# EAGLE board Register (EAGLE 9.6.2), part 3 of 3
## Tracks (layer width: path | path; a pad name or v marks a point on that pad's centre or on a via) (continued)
N$147  (via drill 0.35) (continued)
  Top 0.152: 87.01,49.94 87.01,46.2 87.19,46.03 89.32,46.03 90.03,46.74 90.03,47.27 IC66.3 | 87.01,49.94 89.32,52.25 90.74,52.25 91.27,52.78 91.27,53.49 IC66.13 | v17.84,44.07 17.84,42.47 IC27.11 | v65.49,45.49 68.87,45.49 69.05,45.31 71.89,45.31 75.45,48.87 77.58,48.87 78.3,48.16 78.3,47.45 IC65.3 78.3,47.27 77.76,46.74 v77.76,45.85 | v78.12,51.18 79.54,52.6 79.54,53.49 IC65.13 | v85.41,49.94 87.01,49.94
  Route2 0.152: v17.84,44.07 17.84,42.82 21.4,39.27 25.49,39.27 29.04,42.82 62.83,42.82 v65.49,45.49
  Route3 0.152: v85.41,49.94 79.36,49.94 v78.12,51.18
  Bottom 0.152: v78.12,51.18 78.12,46.2 v77.76,45.85
N$148  (via drill 0.35)
  Top 0.152: v27.09,34.65 26.38,35.36 26.38,36.25 IC111.2 | v97.32,66.12 94.83,66.12 94.12,65.41 94.12,64.69 IC56.11
  Route14 0.152: v27.09,34.65 27.44,34.65 43.98,51.18 50.38,51.18 64.78,65.58 96.79,65.58 v97.32,66.12
N$149  (via drill 0.35)
  Top 0.152: v30.29,34.65 29.93,34.65 29.04,35.53 29.04,36.25 IC111.4 | v80.07,55.98 90.21,55.98 91.45,57.23 91.99,57.23 92.7,57.94 92.7,58.47 IC56.5
  Route3 0.152: v30.29,34.65 46.82,51.18 56.96,51.18 58.2,52.43 62.83,52.43 66.03,55.63 79.72,55.63 v80.07,55.98
N$150  (via drill 0.35)
  Top 0.152: v31.36,34.65 31.36,36.25 IC111.6 | v82.56,61.14 82.56,64.34 IC55.11
  Route14 0.152: v31.36,34.65 37.05,34.65 60.69,58.29 73.85,58.29 76.7,61.14 v82.56,61.14
N$151  (via drill 0.35)
  Top 0.152: v32.6,45.14 32.6,42.47 IC111.10 | v78.3,60.43 79.54,60.43 80.96,59 IC55.5
  Route2 0.152: v32.6,45.14 34.73,47.27 34.73,47.45 48.25,60.96 58.38,60.96 61.05,58.29 76.16,58.29 v78.3,60.43
N$156  (via drill 0.35)
  Top 0.152: v76.87,60.25 75.98,59.36 75.98,58.65 IC55.1 | v93.76,60.25 96.61,60.25 98.92,57.94 98.92,57.4 99.1,57.23 100.16,57.23 100.88,57.94 100.88,58.47 IC58.2
  Route14 0.152: v76.87,60.25 77.41,60.25 77.94,59.72 89.5,59.72 89.67,59.54 93.05,59.54 v93.76,60.25
N$157
  Top 0.152: IC56.15 88.96,64.69 88.96,65.23 90.56,66.83 100.25,66.83 100.88,66.2 100.88,64.69 IC58.13
N$158
  Top 0.152: IC56.1 87.72,58.65 87.72,59.18 90.03,61.49 103.37,61.49 106.03,64.16 106.03,64.52 IC58.9
N$159
  Top 0.152: IC58.6 106.21,58.65 106.21,61.67 107.99,63.45 107.99,65.76 106.57,67.18 78.47,67.18 77.23,65.94 77.23,64.69 IC55.15
N$160
  Top 0.152: IC98.5 44.87,3.71 44.87,4.24 47.18,6.55 62.47,6.55 64.6,8.69 64.6,9.58 IC97.13
N$161  (via drill 0.35)
  Top 0.152: 50.74,48.51 50.74,46.2 50.91,46.03 53.23,46.03 53.94,46.74 53.94,47.27 IC61.3 | 50.74,48.51 55.18,52.96 55.18,53.49 IC61.13 | v22.47,38.2 19.09,38.2 17.84,36.96 17.84,36.42 IC27.4 | v35.45,44.42 35.45,44.96 39.36,48.87 41.31,48.87 42.2,47.98 42.2,47.45 IC60.3 | v42.2,51.18 43.45,52.43 43.45,53.49 IC60.13 | v49.49,48.51 50.74,48.51
  Route2 0.152: v49.49,48.51 44.87,48.51 v42.2,51.18
  Route3 0.152: v22.47,38.2 23.36,38.2 28.69,43.54 34.56,43.54 v35.45,44.42
  Bottom 0.152: v35.45,44.42 v42.2,51.18
N$162  (via drill 0.35)
  Top 0.152: v38.29,31.45 38.29,31.09 34.38,27.18 33.13,27.18 31.53,25.58 31.53,24.87 IC110.6 | v58.56,51.71 58.56,52.25 57.85,52.96 57.85,53.49 IC61.11
  Route3 0.152: v58.56,51.71 v38.29,31.45
N$163  (via drill 0.35)
  Top 0.152: v32.78,32.69 32.78,31.09 IC110.10 | v49.31,45.85 50.56,45.85 50.74,45.67 55.36,45.67 56.43,46.74 56.43,47.27 IC61.5
  Bottom 0.152: v32.78,32.69 32.78,33.58 45.05,45.85 v49.31,45.85
N$164  (via drill 0.35)
  Top 0.152: v29.22,29.31 30.11,30.2 30.11,30.91 IC110.12 | v44.51,51.89 44.87,51.89 45.94,52.96 45.94,53.49 IC60.11
  Route3 0.152: v29.22,29.31 29.22,36.6 v44.51,51.89
N$165
  Top 0.152: IC110.15 26.38,31.09 26.38,31.62 28.69,33.93 31.71,33.93 32.07,34.29 32.07,39.98 33.31,41.22 33.31,48.51 34.38,49.58 43.09,49.58 44.69,47.98 44.69,47.45 IC60.5
N$170
  Top 0.152: IC60.1 39.71,47.27 39.71,46.74 41.31,45.14 55.88,45.14 56.78,46.04 59.42,46.04 60.33,45.14 63,45.14 64.6,46.74 64.6,47.27 IC63.2
N$171
  Top 0.152: IC61.15 52.87,53.67 52.87,54.2 53.94,55.27 63.54,55.27 64.6,54.2 64.6,53.67 IC63.13
N$172
  Top 0.152: IC61.1 51.45,47.45 51.45,47.98 54.47,51 69.41,51 69.94,51.54 69.94,53.49 IC63.9
N$173  (via drill 0.35)
  Top 0.152: v59.09,50.11 59.45,50.47 68.16,50.47 69.76,48.87 69.76,47.45 IC63.6 | v44.51,55.27 42.02,55.27 40.96,54.2 IC60.15
  Route15 0.152: v59.09,50.11 50.03,50.11 45.58,54.56 45.22,54.56 v44.51,55.27
N$174  (via drill 0.35)
  Top 0.152: v85.23,3.53 87.54,3.53 IC99.1 | v50.38,9.04 48.43,9.04 47.71,8.33 46.82,8.33 46.11,9.04 46.11,9.58 IC98.9
  Route2 0.152: v85.23,3.53 61.4,3.53 58.03,6.91 53.94,6.91 51.8,9.04 v50.38,9.04
N$175  (via drill 0.35)
  Top 0.152: v87.01,60.96 87.01,57.23 89.5,57.23 90.03,57.76 90.03,58.47 IC56.3 | IC56.13 91.27,64.52 91.27,63.98 89.5,62.2 88.43,62.2 88.07,62.56 v87.72,62.56 85.41,64.87 85.41,65.94 84.87,66.47 80.96,66.47 79.72,65.23 79.72,64.69 IC55.13 79.54,64.52 79.54,62.74 77.58,60.78 77.58,59.89 78.3,59.18 78.3,58.65 IC55.3 78.3,58.47 78.3,57.76 v76.87,56.34 | v20.87,51.18 19.62,51.18 17.84,52.96 17.84,53.49 IC24.11
  Route3 0.152: v20.87,51.18 24.24,51.18 25.67,52.6 37.76,52.6 37.93,52.43 40.25,52.43 40.6,52.78 62.65,52.78 65.85,55.98 76.52,55.98 v76.87,56.34
  Bottom 0.152: v87.01,60.96 87.01,61.85 v87.72,62.56
N$177  (via drill 0.35)
  Top 0.152: v29.76,21.31 30.11,20.96 30.11,19.71 IC109.12 | v93.97,52.21 v93.96,52.21 93.96,53.54 IC66.11
  Route15 0.152: v29.76,21.31 29.76,21.67 35.27,27.18 46.11,27.18 67.27,48.34 74.21,48.34 78.47,52.6 93.73,52.6 93.97,52.37 v93.97,52.21
N$178  (via drill 0.35)
  Top 0.152: v27.98,17.93 27.44,17.93 26.38,19 26.38,19.53 IC109.15 | v91.81,49.05 92.7,48.16 92.7,47.45 IC66.5
  Route3 0.152: v27.98,17.93 28.87,17.93 63.54,52.6 72.25,52.6 80.61,44.25 80.61,43.71 86.12,38.2 87.19,38.2 88.25,39.27 88.25,45.49 v91.81,49.05
N$179  (via drill 0.35)
  Top 0.152: v26.91,27.36 26.38,26.82 26.38,24.87 IC110.2 | v80.07,51.89 81.14,51.89 82.21,52.96 82.21,53.49 IC65.11
  Route2 0.152: v26.91,27.36 30.65,27.36 45.76,42.47 70.65,42.47 v80.07,51.89
N$180  (via drill 0.35)
  Top 0.152: v33.31,28.96 32.42,28.96 29.04,25.58 29.04,24.87 IC110.4 | v80.07,49.05 80.96,48.16 IC65.5
  Route2 0.152: v33.31,28.96 34.73,30.38 34.73,30.56 41.49,37.31 56.25,37.31 61.05,42.11 72.96,42.11 79.9,49.05 v80.07,49.05
N$185
  Top 0.152: IC65.1 75.98,47.27 75.98,46.56 77.41,45.14 99.28,45.14 100.88,46.74 100.88,47.27 IC68.2
N$186
  Top 0.152: IC66.15 88.96,53.67 88.96,54.2 90.92,56.16 99.28,56.16 100.88,54.56 100.88,53.67 IC68.13
N$187
  Top 0.152: IC66.1 87.72,47.45 87.72,50.11 88.43,50.83 103.9,50.83 106.03,52.96 106.03,53.49 IC68.9
N$188  (via drill 0.35)
  Top 0.152: v103.54,45.67 104.79,45.67 106.03,46.91 106.03,47.27 IC68.6 | v88.96,55.27 77.76,55.27 77.23,54.74 77.23,53.67 IC65.15
  Route2 0.152: v103.54,45.67 102.3,45.67 93.23,54.74 89.5,54.74 v88.96,55.27
N$189  (via drill 0.35)
  Top 0.152: v49.14,7.26 46.65,7.26 44.87,9.04 44.87,9.58 IC98.10 | v85.41,5.66 85.41,8.69 87.01,10.29 87.01,11 87.19,11.18 88.07,11.18 88.79,10.47 88.79,9.75 IC99.13
  Bottom 0.152: v49.14,7.26 50.03,7.26 53.05,4.24 67.63,4.24 67.98,3.89 83.63,3.89 v85.41,5.66
N$190  (via drill 0.35)
  Top 0.152: v77.76,1.4 78.47,0.69 94.65,0.69 97.5,3.53 99.63,3.53 IC100.1 | v40.96,5.31 40.96,6.55 43.45,9.04 43.45,9.58 IC98.11
  Bottom 0.152: v77.76,1.4 58.74,1.4 58.56,1.22 45.05,1.22 v40.96,5.31
N$191  (via drill 0.35)
  Top 0.152: IC98.12 42.22,10.94 42.46,11.18 v50.56,11.18 | v86.12,8.33 87.36,8.33 88.79,6.91 98.74,6.91 100.88,9.04 100.88,9.58 IC100.13
  Route2 0.152: v50.56,11.18 52.69,11.18 56.6,7.26 85.05,7.26 v86.12,8.33
N$192
  Top 0.152: IC98.13 40.96,8.51 35.98,3.53 OUTPUT.4
N$194  (via drill 0.35)
  Top 0.152: IC109.2 v26.35,14.61 | v57.73,43.91 57.73,43.89 57.73,43.59 57.73,42.5 IC71.11
  Route14 0.152: v35.56,20 37.99,22.43 38.56,22.43 55.24,39.1 55.24,41.14 57.73,43.64 v57.73,43.91
  Route15 0.152: v26.35,14.61 31.75,20 v35.56,20
N$195  (via drill 0.35)
  Top 0.152: v32.07,17.93 29.04,14.91 29.04,13.49 IC109.4 | v52.34,38.02 55.36,38.02 56.43,36.96 56.43,36.42 IC71.5
  Route3 0.152: v32.07,17.93 32.07,18.29 35.27,21.49 35.27,23.09 50.2,38.02 v52.34,38.02
N$196  (via drill 0.35)
  Top 0.152: v33.31,16.87 31.53,15.09 31.53,13.49 IC109.6 | v46.29,40.51 46.29,42.11 46.11,42.29 IC70.11
  Route2 0.152: v42.56,38.02 43.8,38.02 v46.29,40.51
  Bottom 0.152: v33.31,16.87 37.22,16.87 41.85,21.49 41.85,37.31 v42.56,38.02
N$197  (via drill 0.35)
  Top 0.152: v36.16,27.89 35.09,26.82 34.02,26.82 33.31,26.11 33.31,22.55 32.78,22.02 32.78,19.71 IC109.10 | v40.96,32.69 42.91,32.69 44.69,34.47 44.69,36.25 IC70.5
  Bottom 0.152: v40.96,32.69 v36.16,27.89
N$202  (via drill 0.35)
  Top 0.152: v64.96,38.56 64.96,36.6 64.78,36.42 IC73.2 | IC70.1 39.69,37.94 v39.53,38.1
  Route3 0.152: v39.53,38.1 48.18,46.75 v50.08,46.75 | v64.96,40.34 64.96,43.67 64.84,43.8 64.84,45.02 v62.51,47.35
  Route15 0.152: v50.08,46.75 61.91,46.75 v62.51,47.35
  Bottom 0.152: v64.96,38.56 v64.96,40.34
N$203
  Top 0.152: IC71.15 52.87,42.47 52.87,43.18 53.94,44.25 56.52,44.25 57.04,44.77 59.17,44.77 59.69,44.25 63.54,44.25 64.6,43.18 64.6,42.47 IC73.13
N$204
  Top 0.152: IC71.1 51.45,36.42 51.45,38.2 52.87,39.62 67.63,39.62 69.76,41.76 69.76,42.29 IC73.9
N$205
  Top 0.152: IC70.15 40.96,43 42.74,44.78 56.2,44.78 56.82,45.4 59.39,45.4 60.01,44.78 69.41,44.78 70.47,43.71 70.47,41.22 69.94,40.69 69.94,36.42 IC73.6
N$206
  Top 0.152: IC98.1 39.54,3.53 38.29,3.53 36.33,1.58 35.27,1.58 33.49,3.35 OUTPUT.3
N$208  (via drill 0.35)
  Top 0.152: v48.07,22.38 48.07,18.29 47.36,17.58 46.82,17.58 44.87,15.62 44.87,13.84 IC108.6 | v98.74,40.51 98.74,42.11 96.96,43.89 94.83,43.89 94.12,43.18 94.12,42.47 IC76.11
  Route2 0.152: v48.07,22.38 57.85,22.38 58.03,22.2 62.12,22.2 71.54,31.62 102.43,31.62 104.08,33.28 104.08,35.17 v98.74,40.51
N$209  (via drill 0.35)
  Top 0.152: v45.76,18.29 45.94,18.47 45.94,19.89 IC108.10 | v92.16,38.02 92.21,38.02 92.71,37.52 IC76.5
  Route15 0.152: v45.76,18.29 64.78,37.31 91.45,37.31 v92.16,38.02
N$210  (via drill 0.35)
  Top 0.152: v43.45,21.67 43.45,20.07 IC108.12 | v77.58,38.56 78.83,38.56 82.21,41.94 82.21,42.29 IC75.11
  Route15 0.152: v43.45,21.67 45.4,21.67 50.74,27 50.74,27.53 61.05,37.85 76.87,37.85 v77.58,38.56
N$211  (via drill 0.35)
  Top 0.152: v39.89,21.67 39.71,21.49 39.71,20.07 IC108.15 | v80.07,38.02 80.07,37.67 80.96,36.78 IC75.5
  Route14 0.152: v39.89,21.67 60.34,42.11 75.45,42.11 79.54,38.02 v80.07,38.02
N$216
  Top 0.152: IC75.1 75.98,36.25 75.98,35.71 77.76,33.93 99.63,33.93 100.88,35.18 100.88,36.25 IC78.2
N$217
  Top 0.152: IC76.15 88.96,42.47 88.96,43 90.21,44.25 99.81,44.25 100.88,43.18 100.88,42.47 IC78.13
N$218
  Top 0.152: IC76.1 87.72,36.42 87.72,36.96 90.03,39.27 103.37,39.27 106.03,41.94 106.03,42.29 IC78.9
N$219  (via drill 0.35)
  Top 0.152: v77.76,40.87 77.23,41.4 77.23,42.29 IC75.15 | v105.14,38.02 106.03,37.14 106.03,36.42 IC78.6
  Route2 0.152: v77.76,40.87 89.32,40.87 89.85,41.4 101.77,41.4 v105.14,38.02
N$220  (via drill 0.35)
  Top 0.152: v52.16,7.62 52.69,8.15 52.69,9.58 IC92.13
  Route2 0.152: v52.16,7.62 50.91,7.62 47.89,4.6 31.89,4.6 30.82,3.53 OUTPUT.2
N$222
  Top 0.152: IC22.15 51.45,20.07 51.45,20.42 53.4,22.38 56.07,22.38 57.14,23.44 57.14,30.38 57.67,30.91 IC81.11
N$223  (via drill 0.35)
  Top 0.152: IC81.5 56.52,23.84 55.94,23.27 v55.89,23.27 | IC108.2 v39.69,12.41
  Route2 0.152: v46.65,16.33 42.38,20.6 42.38,23.62 42.91,24.16 55,24.16 v55.89,23.27
  Route3 0.152: v39.69,12.41 41.14,13.86 41.14,15.56 41.92,16.33 v46.65,16.33
N$224  (via drill 0.35)
  Top 0.152: v46.11,32.69 46.11,31.09 IC80.11 | v58.38,22.91 58.38,20.6 57.85,20.07 IC22.10
  Route2 0.152: v51.45,27.18 54.11,27.18 v58.38,22.91
  Bottom 0.152: v46.11,32.69 51.45,27.36 v51.45,27.18
N$225  (via drill 0.35)
  Top 0.152: IC108.4 42.2,13.84 42.2,12.49 v42.18,12.47 | IC80.5 44.69,24.87 44.69,23.27 44.45,23.02 44.45,22.62 v44.39,22.57
  Route14 0.152: v44.39,22.57 44.39,14.68 v42.18,12.47
N$230  (via drill 0.35)
  Top 0.152: v43.09,23.27 40.78,23.27 39.71,24.33 39.71,24.87 IC80.1 | v64.07,23.09 64.07,23.62 64.6,24.16 64.6,24.87 IC83.2
  Route2 0.152: v43.09,23.27 44.87,23.27 45.58,22.56 46.89,22.56 47.78,21.67 62.65,21.67 v64.07,23.09
N$231
  Top 0.152: IC81.15 52.87,31.09 52.87,31.8 54.83,33.76 63.89,33.76 64.6,33.05 64.6,31.09 IC83.13
N$232  (via drill 0.35)
  Top 0.152: v53.4,27.89 51.45,25.93 51.45,24.87 IC81.1 | v70.29,29.31 70.29,30.56 69.94,30.91 IC83.9
  Route3 0.152: v53.4,27.89 61.76,27.89 62.47,28.6 69.58,28.6 v70.29,29.31
N$233  (via drill 0.35)
  Top 0.152: IC80.15 40.96,29.59 41.23,29.31 v42.56,29.31 | v70.29,26.47 70.29,25.22 69.94,24.87 IC83.6
  Route3 0.152: v42.56,29.31 50.38,29.31 53.23,26.47 v70.29,26.47
N$234  (via drill 0.35)
  Top 0.152: v50.38,3.71 51.27,3.71 IC92.1
  Bottom 0.152: v50.38,3.71 43.62,3.71 41.31,6.02 30.82,6.02 28.33,3.53 OUTPUT.1
N$237  (via drill 0.35)
  Top 0.152: v52.87,12.07 52.51,12.07 51.45,13.13 51.45,13.67 IC22.2 | v95.19,26.47 95.19,28.42 94.12,29.49 94.12,30.91 IC86.11
  Route3 0.152: v52.87,12.07 77.23,12.07 80.25,15.09 91.81,15.09 95.19,18.47 v95.19,26.47
N$238  (via drill 0.35)
  Top 0.152: v54.11,15.44 54.11,13.84 IC22.4 | v92.34,26.47 92.34,26.33 92.71,25.97 IC86.5
  Route3 0.152: v54.11,15.44 54.65,15.44 60.34,21.13 92.7,21.13 93.05,21.49 93.05,25.76 v92.34,26.47
N$239  (via drill 0.35)
  Top 0.152: v64.96,16.15 63.72,16.15 59.98,12.42 57.32,12.42 56.6,13.13 56.6,13.67 IC22.6 | v81.14,29.31 82.21,30.38 82.21,30.91 IC85.11
  Route15 0.152: v64.96,16.15 66.38,16.15 78.83,28.6 80.43,28.6 v81.14,29.31
N$240  (via drill 0.35)
  Top 0.152: v54.47,18.29 55.18,19 55.18,19.89 IC22.12 | v77.58,23.27 79.9,23.27 80.96,24.33 IC85.5
  Route2 0.152: v54.47,18.29 60.87,18.29 63.18,20.6 74.92,20.6 v77.58,23.27
N$245  (via drill 0.35)
  Top 0.152: v78.65,27.18 77.41,27.18 75.98,25.76 75.98,24.87 IC85.1 | v97.5,27.18 99.28,27.18 100.88,25.58 100.88,24.87 IC88.2
  Route2 0.152: v78.65,27.18 88.43,27.18 88.61,27.36 97.32,27.36 v97.5,27.18
N$246
  Top 0.152: IC86.15 88.96,31.09 88.96,31.62 90.74,33.4 99.63,33.4 100.88,32.16 100.88,31.09 IC88.13
N$247  (via drill 0.35)
  Top 0.152: v97.68,23.44 88.43,23.44 87.72,24.16 87.72,24.87 IC86.1 | v106.21,27.71 106.21,28.07 109.05,30.91 109.05,32.16 108.7,32.51 106.92,32.51 106.21,31.8 106.21,31.09 IC88.9
  Route2 0.152: v97.68,23.44 99.63,23.44 101.94,25.76 106.39,25.76 106.92,26.29 106.92,27 v106.21,27.71
N$248  (via drill 0.35)
  Top 0.152: v79.36,29.31 78.3,29.31 77.23,30.38 77.23,30.91 IC85.15 | v106.21,26.65 106.21,24.87 IC88.6
  Route2 0.152: v79.36,29.31 80.07,29.31 81.5,27.89 104.97,27.89 v106.21,26.65
NUMBER1  (via drill 0.35)
  Top 0.152: v82.38,26.47 82.38,24.87 IC85.6 | v83.63,38.02 83.27,37.67 83.1,37.67 82.38,36.96 82.38,36.42 IC75.6 | v82.21,49.05 82.21,47.45 IC65.6 | v83.27,60.43 82.38,59.54 82.38,58.65 IC55.6 | v82.38,71.98 82.38,70.38 IC45.6 | v82.38,80.34 82.38,81.94 IC35.6 | IC25.6 82.21,93.14 v82.21,94.74 82.56,95.1 v82.56,97.05 | v82.38,106.3 82.38,104.7 IC12.6 | IC108.5 43.62,13.84 43.62,15.09 46.82,18.29 v47,18.29 | IC80.6 46.11,24.87 46.11,23.44 v45.94,23.27 | v45.94,38.02 45.94,36.42 IC70.6 | v53.4,18.29 54.11,17.58 54.83,17.58 56.43,19.18 56.43,19.89 IC22.11 | v32.78,28.07 30.29,25.58 30.29,24.87 IC110.5 | v34.02,21.31 34.02,19.71 IC109.9 | IC110.14 27.62,31.62 28.69,32.69 v30.47,32.69 | v33.85,39.45 33.85,42.29 IC111.9 | v40.96,21.67 IC108.14 | IC112.14 27.62,52.07 v26.02,50.47 | v29.4,45.67 30.11,46.38 30.11,47.27 IC112.5 | 35.09,64.69 37.93,64.69 41.14,67.89 44.16,67.89 45.94,69.67 45.94,70.21 IC40.6 46.04,71.6 46.88,72.44 v48.62,72.44 | 35.09,64.69 34.02,64.69 IC113.9 | v47,50.29 46.11,49.4 46.11,47.45 IC60.6 | v47.36,56.69 46.11,57.94 46.11,58.47 IC50.6 | v46.11,80.16 46.11,81.94 IC30.6 | IC114.14 27.62,74.12 26.56,73.05 26.56,72.34 27.27,71.63 29.4,71.63 30.11,70.92 | 30.11,70.92 30.11,70.38 IC114.5 30.11,70.92 | v33.31,94.74 32.6,95.45 31.1,95.45 30.29,94.65 30.29,93.14 IC116.5 | IC20.6 45.94,93.14 45.94,94.39 44.69,95.63 39.54,95.63 37.93,94.03 v37.58,94.03 | v33.85,89.76 33.85,88.16 IC115.9 | IC116.14 27.62,100.22 28.37,100.97 v31.18,100.97 | v42.74,102.03 44.69,102.03 45.94,103.28 45.94,104.52 IC10.6 | v34.02,108.97 34.02,110.57 IC117.9 | 30.11,70.92 33.13,73.94 33.67,73.94 v34.38,74.65
  Top 0.152: v35.09,66.65 35.09,64.69
  Route2 0.152: v82.38,26.47 78.83,26.47 73.32,20.96 56.07,20.96 v53.4,18.29
  Route14 0.152: v47,18.29 47,19.56 45.94,20.62 v45.94,23.27 | v33.31,94.74 36.86,94.74 v37.58,94.03
  Route15 0.152: v26.02,50.47 26.02,48.87 29.22,45.67 | 29.22,45.67 33.85,41.05 v33.85,39.45 | 29.22,45.67 v29.4,45.67 | v45.94,23.27 44.16,23.27 43.27,22.38 41.67,22.38 v40.96,21.67 | v45.94,38.02 45.94,39.09 47,40.16 v47,50.29 | v82.38,80.34 85.08,77.64 85.08,74.68 v82.38,71.98
  Bottom 0.152: 83.81,27.89 84.16,28.25 84.16,37.49 v83.63,38.02 | 83.81,27.89 v82.38,26.47 | 83.81,27.89 82.21,29.49 v82.21,49.05 82.21,51.54 83.27,52.6 v83.27,60.43 83.27,61.49 82.38,62.38 v82.38,71.98 | v82.21,94.74 82.21,80.52 v82.38,80.34 | v82.38,106.3 82.38,97.23 v82.56,97.05 | v45.94,38.02 45.94,33.58 45.4,33.05 45.4,29.49 46.11,28.78 46.11,23.44 v45.94,23.27 | v47,18.29 v53.4,18.29 | v34.02,21.31 34.02,22.38 | 34.02,22.38 34.02,26.29 32.78,27.53 v32.78,28.07 32.6,28.25 32.6,30.02 30.47,32.16 v30.47,32.69 33.85,36.07 v33.85,39.45 | v40.96,21.67 40.25,22.38 34.02,22.38 | v47,50.29 47,50.65 47.89,51.54 47.89,56.16 v47.36,56.69 47.36,66.83 48.6,68.07 48.6,72.45 | 34.02,102.03 32.25,102.03 v31.18,100.97 31.18,97.41 33.31,95.28 v33.31,94.74 33.85,94.21 v33.85,89.76 33.85,80.34 34.38,79.81 v34.38,74.65 35.09,73.94 v35.09,66.65 | 34.02,102.03 v42.74,102.03 | 34.02,102.03 v34.02,108.97 32.25,110.74 32.25,115.37 31.18,116.43 30.47,116.43 29.4,115.37 28.33,115.37 NUMBER.1 | 48.6,72.45 48.6,75.18 46.11,77.67 v46.11,80.16 | v48.62,72.44 48.6,72.45
NUMBER2  (via drill 0.35)
  Top 0.152: v47.36,100.97 47.36,99.37 IC20.10 | v47.36,106.3 47.36,110.57 IC10.10 | v29.93,112.88 30.65,112.17 34.38,112.17 38.29,108.26 39.53,108.26 39.83,108.56 v40.8,108.56 | v47.36,32.69 47.36,31.09 IC80.10 | v47.36,38.91 47.36,42.29 IC70.10 | v46.65,61.32 46.65,63.98 47.18,64.52 IC50.10 | IC60.10 47.18,53.49 v47.18,51.89 45.58,51.89 44.16,50.47 v39.36,50.47 | v47.89,74.83 47.36,75.36 47.36,76.25 IC40.10 | v47.18,86.56 47.18,88.16 IC30.10 | v83.45,29.31 83.45,30.91 IC85.10 | v82.92,38.73 82.92,41.76 83.45,42.29 IC75.10 | v83.45,51.71 83.45,53.49 IC65.10 | v83.63,62.92 83.63,64.52 IC55.10 | v83.63,74.65 83.63,76.25 IC45.10 | v83.63,86.56 83.63,88.16 IC35.10 | v83.27,94.74 83.45,94.92 v83.45,97.59 83.45,99.19 IC25.10 | v83.45,108.43 83.45,110.57 IC12.10 | IC116.3 27.62,94.17 28.19,94.74 v28.51,94.74 | v26.91,95.45 27.46,95.45 29.16,97.15 30.49,97.15 31.36,98.02 31.36,99.19 IC116.11 | 57.85,15.44 57.85,18.11 58.92,19.18 58.92,19.89 IC22.9 | 57.85,15.44 57.85,13.84 IC22.7 | IC113.7 32.6,58.47 32.6,56.69 31.53,55.63 31.53,53.67 IC112.11 31.36,53.49 v31.36,51.89 | 29.04,28.07 31.36,30.38 31.36,30.91 IC110.11 31.53,31.09 31.53,32.51 32.6,33.58 32.6,36.25 IC111.7 | 29.04,28.07 27.62,26.65 IC110.3 27.62,24.33 29.93,22.02 v31.18,22.02 | v32.6,15.09 32.6,13.49 IC109.7 | v27.62,45.67 IC112.3 | 29.04,28.07 v27.8,29.31 | v27.62,68.61 IC114.3 | v27.27,72.7 28.33,72.7 31.36,75.72 31.36,76.25 IC114.11 | v27.98,80.16 31.36,80.16 32.6,81.41 32.6,81.94 IC115.7 | v42.91,15.44 44.69,17.22 44.69,19.89 IC108.11 | v56.07,15.44 57.85,15.44 | IC117.7 v32.7,105.89
  Route2 0.152: v42.91,15.44 32.96,15.44 v32.6,15.09 | v31.36,51.89 31.36,49.4 v27.62,45.67
  Route3 0.152: v56.07,15.44 55.18,15.44 54.47,14.73 43.62,14.73 v42.91,15.44
  Route14 0.152: v47.36,100.97 47.36,86.74 v47.18,86.56 | v32.7,105.89 29.93,108.66 v29.93,112.88
  Route15 0.152: v47.36,38.91 47.36,49.58 47.71,49.94 47.71,51.36 v47.18,51.89 | v28.51,94.74 28.51,92.08 29.22,91.36 29.22,84.61 27.98,83.36 v27.98,80.16 | v83.45,29.31 82.21,29.31 68.34,15.44 v56.07,15.44 | v40.8,108.56 45.1,108.56 v47.36,106.3
  Bottom 0.152: v47.36,106.3 v47.36,100.97 | v29.93,112.88 28.16,112.88 25.84,115.19 NUMBER.2 | v47.36,38.91 v47.36,32.69 | v47.18,51.89 47.18,55.8 46.65,56.34 v46.65,61.32 46.65,66.65 47.89,67.89 v47.89,74.83 45.4,77.32 45.4,80.52 47.18,82.3 v47.18,86.56 | v83.45,29.31 83.45,37.14 82.92,37.67 v82.92,38.73 83.45,39.27 v83.45,51.71 83.99,52.25 83.99,60.78 83.63,61.14 v83.63,62.92 v83.63,74.65 v83.63,86.56 83.27,86.92 v83.27,94.74 | v83.45,97.59 v83.45,108.43 | v28.51,94.74 27.62,94.74 v26.91,95.45 | v32.6,15.09 32.6,16.33 31.18,17.76 v31.18,22.02 | v27.8,29.31 26.38,30.73 26.38,35.89 27.62,37.14 v27.62,45.67 v27.62,68.61 27.27,68.96 v27.27,72.7 27.27,73.94 27.98,74.65 v27.98,80.16 | v39.36,50.47 32.78,50.47 v31.36,51.89
NUMBER3  (via drill 0.35)
  Top 0.152: 37.76,14.91 37.93,15.09 40.72,15.09 40.96,14.85 IC108.3 | 37.76,14.91 34.59,11.75 30.84,11.75 30.29,12.3 30.29,13.31 IC109.5 | 37.76,14.91 37.76,21.13 38.32,21.69 38.32,23.06 v38.29,23.09 | v27.62,21.31 IC109.14 | IC111.14 27.62,41.94 26.56,40.87 v26.56,39.27 27.8,39.27 30.11,36.96 30.11,36.42 IC111.5 | v34.02,27.89 34.02,30.91 IC110.9 | IC113.14 27.62,63.45 v26.73,62.56 | v26.56,108.97 30.11,105.41 30.11,104.7 IC117.5 | 33.85,53.67 33.92,53.6 | 33.92,53.6 IC112.9 | 30.11,83.72 30.11,84.03 27.62,86.52 IC115.14 | 30.11,83.72 30.11,82.12 IC115.5 | v32.96,74.65 33.85,75.54 33.85,76.25 IC114.9 | 30.11,83.72 v31.18,83.72 | v34.91,98.3 34.02,99.19 IC116.9 | v32.6,61.85 32.58,61.83 31.87,61.83 30.13,60.09 30.13,58.55 IC113.5 30.29,58.47 30.29,56.52 30.09,56.32 27.21,56.32 v26.73,55.84 | v94.12,26.47 94.12,24.87 IC86.6 | v94.12,34.65 94.12,36.25 IC76.6 | v94.12,49.05 94.12,47.45 IC66.6 | v94.12,56.87 94.12,58.47 IC56.6 | v94.12,71.98 94.12,70.38 IC46.6 | v94.12,83.72 94.12,82.12 IC36.6 | IC26.6 93.96,93.15 93.96,94.41 v94.3,94.74 | v94.12,106.3 94.12,104.7 IC16.6 | IC22.5 55.36,13.84 55.36,16.03 55.84,16.51 56.67,16.51 v56.83,16.67 | 57.67,24.87 IC81.6 57.85,24.87 v57.85,29.31 | v58.03,38.02 57.85,37.85 57.85,36.42 IC71.6 | v58.03,49.05 58.03,47.62 57.85,47.45 IC61.6 | v57.85,60.25 57.85,58.65 IC51.6 | v57.85,71.98 57.85,70.38 IC41.6 | v57.85,80.16 57.85,81.94 IC31.6 | v57.85,94.74 57.85,93.14 IC21.6 | v55.89,106.12 56.78,106.12 57.67,105.23 57.67,104.7 IC11.6 | IC108.9 v47.31,21.12 v47.3,21.12 | v34.77,53.66 34.71,53.6 33.92,53.6
  Route2 0.152: v38.29,23.09 39,23.09 44.51,28.6 57.14,28.6 v57.85,29.31
  Route3 0.152: v34.02,27.89 27.62,21.49 v27.62,21.31 | v26.73,55.84 28.14,55.84 30.48,53.5 34.61,53.5 v34.77,53.66
  Route15 0.152: v26.56,108.97 26.56,106.66 v34.91,98.3 | v94.12,71.98 94.12,71.74 93.17,70.8 59.04,70.8 v57.85,71.98 | v47.3,21.12 46.72,20.53 39.78,20.53 38.28,22.03 38.28,23.08 v38.29,23.09 | v57.85,29.31 57.85,23.31 57.72,23.18 57.72,17.56 v56.83,16.67
  Bottom 0.152: v27.62,21.31 27.62,28.42 26.02,30.02 26.02,38.73 v26.56,39.27 26.73,39.45 v26.73,55.84 26.73,55.88 25.88,55.88 25.56,56.2 25.56,58.58 26.73,59.75 v26.73,62.56 | v38.29,23.09 38.29,23.62 v34.02,27.89 | v26.56,108.97 26.56,111.81 23.18,115.19 NUMBER.3 | v31.18,83.72 32.96,81.94 v32.96,74.65 32.96,67.72 34.73,65.94 | v34.91,98.3 34.91,81.41 35.8,80.52 35.8,66.29 35.45,65.94 34.73,65.94 | v32.6,61.85 32.6,63.81 34.73,65.94 | v94.12,26.47 v94.12,34.65 v94.12,49.05 94.12,51.28 94.77,51.93 94.77,54.11 94.12,54.77 v94.12,56.87 94.48,57.23 94.48,60.6 94.12,60.96 v94.12,71.98 94.12,74.47 94.83,75.18 94.83,80.7 94.12,81.41 v94.12,83.72 94.3,83.9 v94.3,94.74 94.12,94.92 v94.12,106.3 | v55.89,106.12 55.89,109.32 56.25,109.68 56.96,109.68 57.85,108.79 v57.85,94.74 57.85,87.27 58.2,86.92 58.2,80.52 v57.85,80.16 v57.85,71.98 v57.85,60.25 57.85,49.23 v58.03,49.05 58.03,47.94 59.69,46.28 59.69,41.35 58.03,39.69 v58.03,38.02 57.85,37.85 v57.85,29.31
NUMBER4  (via drill 0.35)
  Top 0.152: v95.36,29.31 95.36,30.91 IC86.10 | v95.36,40.51 95.36,42.29 IC76.10 | v95.36,51.54 95.36,53.49 IC66.10 | v95.36,62.92 95.36,64.52 IC56.10 | v95.36,74.65 95.36,76.25 IC46.10 | v95.36,86.56 95.36,88.16 IC36.10 | v95.19,97.59 95.19,99.19 IC26.10 | 95.36,111.45 95.36,110.74 IC16.10 95.36,111.45 | 95.36,111.45 96.08,112.17 96.96,112.17 97.14,111.99 v97.14,108.43 | IC113.3 27.62,60.25 31.36,63.98 31.36,64.52 IC113.11 31.53,64.69 31.53,65.41 32.6,66.47 32.6,70.21 IC114.7 32.78,70.38 32.78,71.09 v33.67,71.98 | IC115.3 27.62,83.72 24.07,87.27 24.07,89.92 | 24.07,89.92 24.07,106.12 24.96,107.01 | 24.96,107.01 25.67,107.01 27.62,105.05 IC117.3 | 30.82,89.41 30.47,89.76 v28.51,89.76 | 30.82,89.41 31.36,88.88 31.36,88.16 IC115.11 | 24.07,89.92 v24.16,89.92 | v32.25,94.74 32.6,94.39 32.6,93.14 IC116.7 | 30.82,89.41 v31.36,89.94 | v23.53,108.97 23.53,108.43 24.96,107.01 | IC109.3 27.62,15.27 31.36,19 31.36,19.53 IC109.11 31.53,19.71 31.53,21.31 32.6,22.38 v32.6,23.27 32.6,24.87 IC110.7 | 31.89,46.03 30.82,46.03 29.76,44.96 25.84,44.96 24.42,43.54 24.42,40.34 27.62,37.14 IC111.3 27.62,35.53 v28.51,34.65 | 31.89,46.03 32.6,46.74 32.6,47.27 IC112.7 | 31.89,46.03 31.89,44.96 31.53,44.6 31.53,42.47 IC111.11 | v45.94,15.44 45.94,13.84 IC108.7 | 51.63,15.44 v48.07,15.44 | 51.63,15.44 52.69,14.38 52.69,13.84 IC22.3 | 51.63,15.44 52.69,16.51 52.69,19.89 IC22.14 | v59.09,32.69 59.09,31.09 IC81.10 | v60.69,40.69 60.69,41.05 61.05,41.4 61.05,43.54 60.69,43.89 59.98,43.89 59.09,43 59.09,42.47 IC71.10 | v59.63,51.71 59.09,52.25 59.09,53.49 IC61.10 | v59.63,62.92 59.09,63.45 59.09,64.52 IC51.10
  Top 0.152: v59.09,74.65 59.09,76.25 IC41.10 | v58.92,86.56 58.92,88.16 IC31.10 | v58.92,97.59 58.92,99.19 IC21.10 | v58.92,112.34 58.92,110.74 IC11.10 | v94.48,112.34 95.36,111.45
  Route14 0.152: v48.07,15.44 48.07,16.33 47.89,16.51 47.89,20.78 59.09,31.98 v59.09,32.69
  Route15 0.152: v32.6,23.27 36.09,23.27 43.92,15.44 v45.94,15.44 | v33.67,71.98 35.8,71.98 39.36,75.54 58.2,75.54 v59.09,74.65
  Bottom 0.152: v95.36,29.31 v95.36,40.51 v95.36,51.54 v95.36,62.92 v95.36,74.65 v95.36,86.56 95.19,86.74 v95.19,97.59 95.19,102.03 97.14,103.99 v97.14,108.43 | v28.51,89.76 28.35,89.92 v24.16,89.92 | v32.25,94.74 32.25,90.83 v31.36,89.94 33.31,87.99 33.31,80.34 33.67,79.98 v33.67,71.98 | v23.53,108.97 20.69,111.81 20.69,115.19 NUMBER.4 | v32.6,23.27 32.6,27.18 31.53,28.25 31.53,30.56 28.51,33.58 v28.51,34.65 | v48.07,15.44 v45.94,15.44 | v59.09,32.69 59.09,39.09 v60.69,40.69 60.34,41.05 60.34,49.94 59.63,50.65 v59.63,51.71 v59.63,62.92 59.09,63.45 v59.09,74.65 58.56,75.18 58.56,80.7 58.92,81.05 v58.92,86.56 v58.92,97.59 58.92,111.99 | v94.48,112.34 73.03,112.34 71.96,111.28 68.81,111.28 68.1,111.99 58.92,111.99 | 58.92,111.99 v58.92,112.34
O0  (via drill 0.35)
  Top 0.152: v85.41,21.84 87.9,21.84 88.25,21.49 88.25,19 88.43,18.82 90.56,18.82 91.27,19.53 91.27,20.07 IC91.11 | v66.74,23.27 66.74,23.62 66.21,24.16 66.21,24.87 IC83.3
  Route3 0.152: v85.41,21.84 84.52,22.73 83.27,22.73 83.1,22.55 70.83,22.55 70.12,23.27 v66.74,23.27
O1
  Top 0.152: IC94.11 67.45,20.24 67.45,24.87 IC83.4
O2
  Top 0.152: IC97.11 67.45,9.75 67.45,10.47 69.05,12.07 75.63,12.07 76.52,12.95 76.52,16.69 75.45,17.76 74.56,17.76 71.89,20.42 71.89,21.49 69.94,23.44 69.41,23.44 69.23,23.62 69.23,30.38 68.69,30.91 IC83.10
O3  (via drill 0.35)
  Top 0.152: v86.12,7.26 86.83,6.55 100.88,6.55 103.37,9.04 103.37,9.58 IC100.11 | v67.63,29.31 67.63,30.73 67.45,30.91 IC83.11
  Route14 0.152: v86.12,7.26 80.78,7.26 72.78,15.27 72.78,22.91 67.63,28.07 v67.63,29.31
P0
  Top 0.152: IC91.12 90.21,20.24 90.21,20.78 91.99,22.55 101.41,22.55 102.12,23.27 102.12,24.87 IC88.3
P1  (via drill 0.35)
  Top 0.152: v66.74,22.02 66.21,21.49 66.21,20.24 IC94.12 | v105.14,29.31 105.14,28.42 103.54,26.82 103.54,24.87 IC88.4
  Route2 0.152: v66.74,22.02 68.16,22.02 76.16,30.02 104.43,30.02 v105.14,29.31
P2  (via drill 0.35)
  Top 0.152: v65.67,11.35 66.03,11 66.03,9.75 IC97.12 | v105.32,32.69 105.32,31.62 104.79,31.09 IC88.10
  Route2 0.152: v65.67,11.35 66.56,11.35 76.34,21.13 97.85,21.13 102.12,25.4 106.57,25.4 107.28,26.11 107.28,30.73 v105.32,32.69
P3  (via drill 0.35)
  Top 0.152: v101.59,12.42 102.12,11.89 102.12,9.75 IC100.12 | v101.94,26.47 101.94,28.96 103.37,30.38 103.37,30.91 IC88.11
  Bottom 0.152: v101.59,12.42 101.59,20.96 102.12,21.49 102.12,26.29 v101.94,26.47
R  (via drill 0.35)
  Top 0.152: IC17.8 21.58,64.87 v21.58,63.27 20.47,62.16 16.73,62.16 14.83,60.26 13.97,60.26 | IC13.1 13.93,70.21 13.93,67.94 13.22,67.23 13.22,60.69 13.65,60.26 13.97,60.26 | 20.69,41.05 21.58,41.94 21.58,42.29 IC27.8 | 20.69,41.05 19.44,39.8 16.95,39.8 14.11,36.96 14.11,36.42 IC27.1 | v14.11,83.72 14.11,82.12 IC19.8 | v14.11,89.76 14.11,92.96 IC15.8 | v13.93,15.44 13.93,13.49 IC32.1 | IC29.1 13.97,23.23 v14.29,22.91 14.97,22.23 20.27,22.23 v21.53,20.97 21.53,19.65 IC32.8 | v21.4,29.31 21.58,29.49 21.58,30.91 IC29.8 | v19.44,45.31 15.53,45.31 14.11,46.74 14.11,47.27 IC24.1 | v21.58,51.89 21.58,53.49 IC24.8 | v21.58,74.65 21.58,76.25 IC13.8 | v21.58,84.61 21.58,87.99 IC19.1 | v23.16,86.23 23.32,86.39 23.32,98.03 22.07,99.28 IC15.1 21.59,100.95 22.29,101.64 v22.29,109.14 | v21.04,40.69 20.69,41.05 | 13.97,60.26 IC17.1
  Route15 0.152: v14.11,83.72 15.18,83.72 16.07,84.61 v21.58,84.61
  Bottom 0.152: v14.11,89.76 v14.11,83.72 | v13.93,15.44 13.93,22.55 v14.29,22.91 | 20.15,39.8 21.4,38.56 v21.4,29.31 20.29,28.2 20.29,26.19 21.53,24.96 v21.53,20.97 | 20.15,39.8 19.44,40.51 v19.44,45.31 21.58,47.45 v21.58,51.89 v21.58,63.27 v21.58,74.65 v21.58,84.61 23.16,86.19 v23.16,86.23 | v22.29,109.14 18.2,113.23 18.2,115.19 R.1 | 20.15,39.8 v21.04,40.69
W  (via drill 0.35)
  Top 0.152: v19.31,83.4 19.27,83.36 19.27,82.12 IC19.12 | IC15.12 19.09,92.96 19.09,91.88 18.26,91.05 v14.95,91.05 | IC24.5 18.91,47.45 18.91,49.23 16.6,51.54 16.6,53.49 IC24.12 16.42,53.67 16.42,54.92 v16.07,55.27 | IC17.12 16.6,65.05 16.6,65.94 17.3,66.64 v17.3,67.31 | IC32.12 16.51,18.42 16.38,18.29 v16.38,18.14 | 16.07,27.18 16.07,28.6 16.42,28.96 16.42,30.91 IC29.12 | 16.07,27.18 v16.07,26.47 | v12.59,15.52 12.59,13.06 14.64,11 18.2,11 18.91,11.71 18.91,13.31 IC32.5 | 16.07,27.18 18.38,27.18 18.91,26.65 18.91,24.87 IC29.5 | v16.07,34.47 17.84,34.47 18.91,35.53 18.91,36.25 IC27.5 | v15.89,40.87 16.42,41.4 16.42,42.29 IC27.12 | v16.07,56.87 16.42,56.52 18.2,56.52 18.91,57.23 18.91,58.83 IC17.5 | v15.53,73.94 16.42,74.83 16.42,76.25 IC13.12 | v14.82,84.43 16.42,86.03 16.42,87.99 IC19.5 | v16.24,97.59 16.42,97.77 16.42,99.19 IC15.5 | v16.42,102.92 16.42,104.52 IC34.3 | IC13.5 19.07,70.25 v19.07,68.83
  Route2 0.152: v19.07,68.83 18.69,68.45 v15.39,68.45 16.53,67.31 v17.3,67.31
  Route14 0.152: v12.59,15.52 12.59,15.61 15.11,18.14 v16.38,18.14 16.38,19.84 15.43,20.8 15.43,25.83 v16.07,26.47 | v14.82,84.43 18.28,84.43 v19.31,83.4
  Bottom 0.152: v16.07,26.47 14.47,28.07 14.47,30.02 16.07,31.62 v16.07,34.47 15.89,34.65 v15.89,40.87 14.64,42.11 14.64,51.89 16.07,53.31 v16.07,55.27 v16.07,56.87 15.53,57.4 15.53,68.45 | 15.53,68.45 15.53,68.61 15.19,68.61 14.42,69.37 14.42,72.83 v15.53,73.94 13.69,73.94 13.34,74.3 13.34,78.9 14.82,80.39 v14.82,84.43 14.82,91.05 | 14.82,91.05 14.82,96.16 v16.24,97.59 16.42,97.77 v16.42,102.92 | 15.53,68.45 v15.39,68.45 | 14.82,91.05 v14.95,91.05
